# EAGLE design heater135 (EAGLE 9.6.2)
DATABASE: Z:\Eigene Dateien\Anwendungsdaten\Eagle\partdb\exp.txt
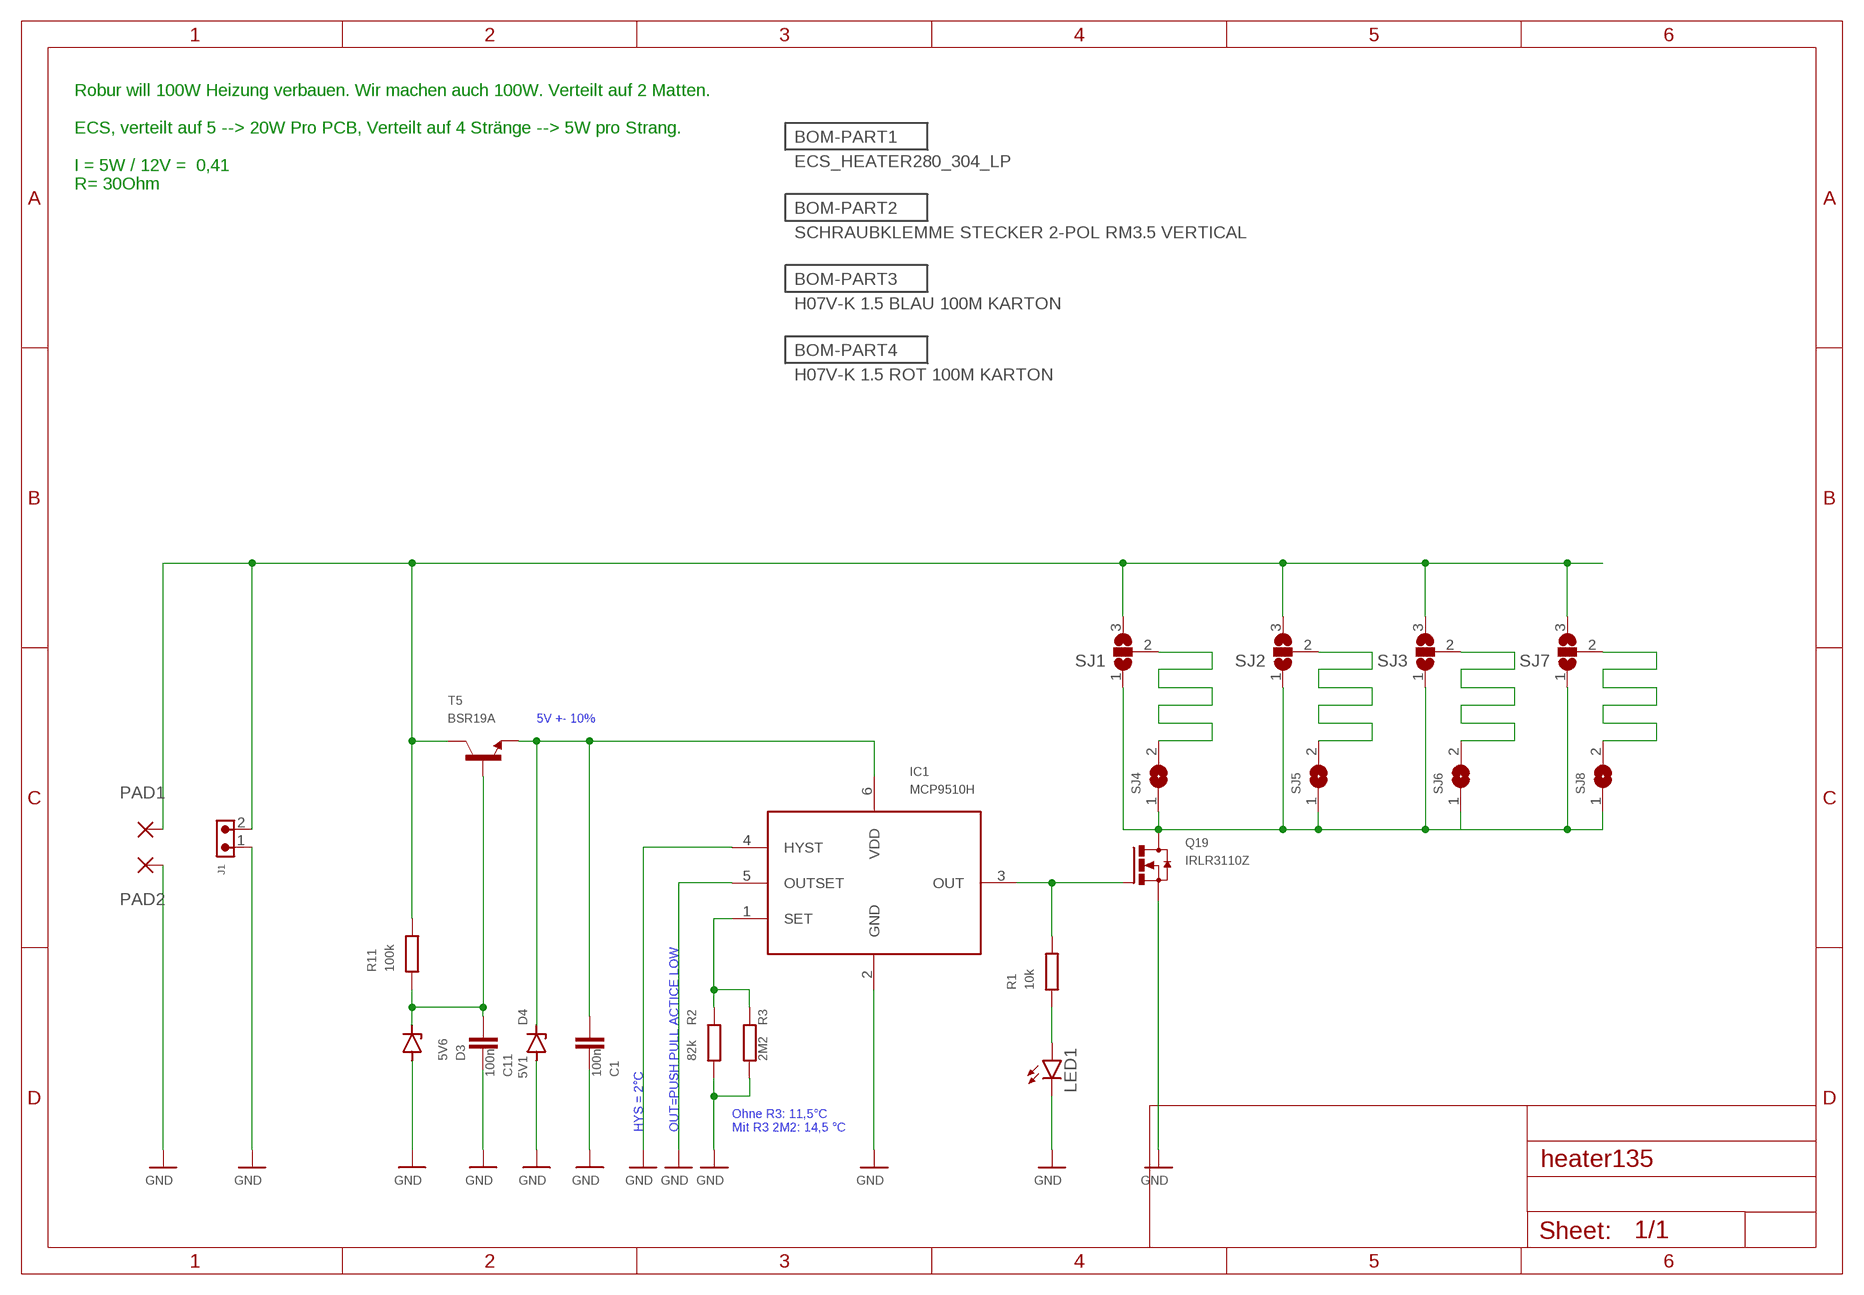
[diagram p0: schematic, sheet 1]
BOM-PART1 (BOM-PART): BOM: INCLUDE; PARTNO: PT055; QTY: 1
BOM-PART2 (BOM-PART): BOM: INCLUDE; PARTNO: CON181; QTY: 1
BOM-PART3 (BOM-PART): BOM: INCLUDE; QTY: 1
BOM-PART4 (BOM-PART): BOM: INCLUDE; QTY: 1

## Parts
C1  100n  C-EUC0603  [C0603]
C11  100n  C-EUC0603  [C0603]
D3  5V6  ZENER-DIODESOD80C  [SOD80C]
D4  5V1  ZENER-DIODESOD80C  [SOD80C]
IC1  MCP9510H  MCP9509  [SOT23-6]
J1  691322110002  [691322110002]
LED1  LEDSML0603  [SML0603]
PAD1  3,81/1,4  [3,81/1,4]
PAD2  3,81/1,4  [3,81/1,4]
Q19  IRLR3110Z  IRFR2607  [D-PACK]
R1  10k  R-EU_R0603  [R0603]
R2  82k  R-EU_R0603  [R0603]
R3  2M2  R-EU_R0603  [R0603]
R11  100k  R-EU_R0603  [R0603]
SJ1  SJ2W  [SJ_2]
SJ2  SJ2W  [SJ_2]
SJ3  SJ2W  [SJ_2]
SJ4  SJ  [SJ]
SJ5  SJ  [SJ]
SJ6  SJ  [SJ]
SJ7  SJ2W  [SJ_2]
SJ8  SJ  [SJ]
T5  BSR19A  MMBT2222ALT1-NPN-SOT23-BEC  [SOT23-BEC]

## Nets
+UB: J1.2 PAD1.1(P) R11.2 SJ1.3 SJ2.3 SJ3.3 SJ7.3 T5.C
GND: C1.2 C11.2 D3.A D4.A IC1.2(GND) IC1.4(HYST) IC1.5(OUTSET) J1.1 LED1.C PAD2.1(P) Q19.3(S) R2.1 R3.1
N$1: IC1.3(OUT) Q19.1(G) R1.2
N$2: SJ1.2 SJ4.2
N$3: C11.1 D3.C R11.1 T5.B
N$4: IC1.1(SET) R2.2 R3.2
N$5: C1.1 D4.C IC1.6(VDD) T5.E
N$6: LED1.A R1.1
N$7: SJ2.2 SJ5.2
N$8: SJ3.2 SJ6.2
N$9: SJ7.2 SJ8.2
N$11: Q19.4(D) SJ1.1 SJ2.1 SJ3.1 SJ4.1 SJ5.1 SJ6.1 SJ7.1 SJ8.1

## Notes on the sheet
- Robur will 100W Heizung verbauen. Wir machen auch 100W. Verteilt auf 2 Matten.
  
  ECS, verteilt auf 5 --> 20W Pro PCB, Verteilt auf 4 Stränge --> 5W pro Strang.
  
  I = 5W / 12V =  0,41
  R= 30Ohm
- 5V +- 10%
- HYS = 2°C | OUT=PUSH PULL ACTICE LOW
- Ohne R3: 11,5°C
  Mit R3 2M2: 14,5 °C

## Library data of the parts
C1 C11 = rcl:C-EU: CAPACITOR, European symbol; PARTNO: C067; SPICEPREFIX: C
D3 = diode:ZENER-DIODE: Z-Diode; PARTNO: D013
D4 = diode:ZENER-DIODE: Z-Diode; PARTNO: D012
IC1 = mcp9509:MCP9509; PARTNO: IC333
J1 = Wurth_Connectors_WR-TBL Pluggable Connector:691322110002: WR-TBL Serie 3221 - 3.50 mm Horizontal PCB Header; DATASHEET-URL: https://www.we-online.com/catalog/datasheet/691322110002.pdf; IR-UL: 10A; IR-VDE: 10.5A; MOUNT: THT; PART-NUMBER: 691322110002; PARTNO: CON212; PINS: 2; PITCH: 3.5mm; TYPE: Horizontal; WORKING-VOLTAGE-UL: 300V (AC); WORKING-VOLTAGE-VDE: 300V (AC)
LED1 = led:LED: LED; PARTNO: D078
PAD1 PAD2 = wirepad:3,81/1,4: THROUGH-HOLE PAD
Q19 = IRFR2607:IRFR2607; PARTNO: T086
R1 = rcl:R-EU_: RESISTOR, European symbol; PARTNO: R221; SPICEPREFIX: R
R2 = rcl:R-EU_: RESISTOR, European symbol; PARTNO: R243; SPICEPREFIX: R
R3 = rcl:R-EU_: RESISTOR, European symbol; PARTNO: R277; SPICEPREFIX: R
R11 = rcl:R-EU_: RESISTOR, European symbol; PARTNO: R245; SPICEPREFIX: R
SJ1-SJ3 SJ7 = jumper:SJ2W: SMD solder JUMPER
SJ4-SJ6 SJ8 = jumper:SJ: SMD solder JUMPER
T5 = transistor-neu-to92:*-NPN-: NPN Transistror; PARTNO: T056

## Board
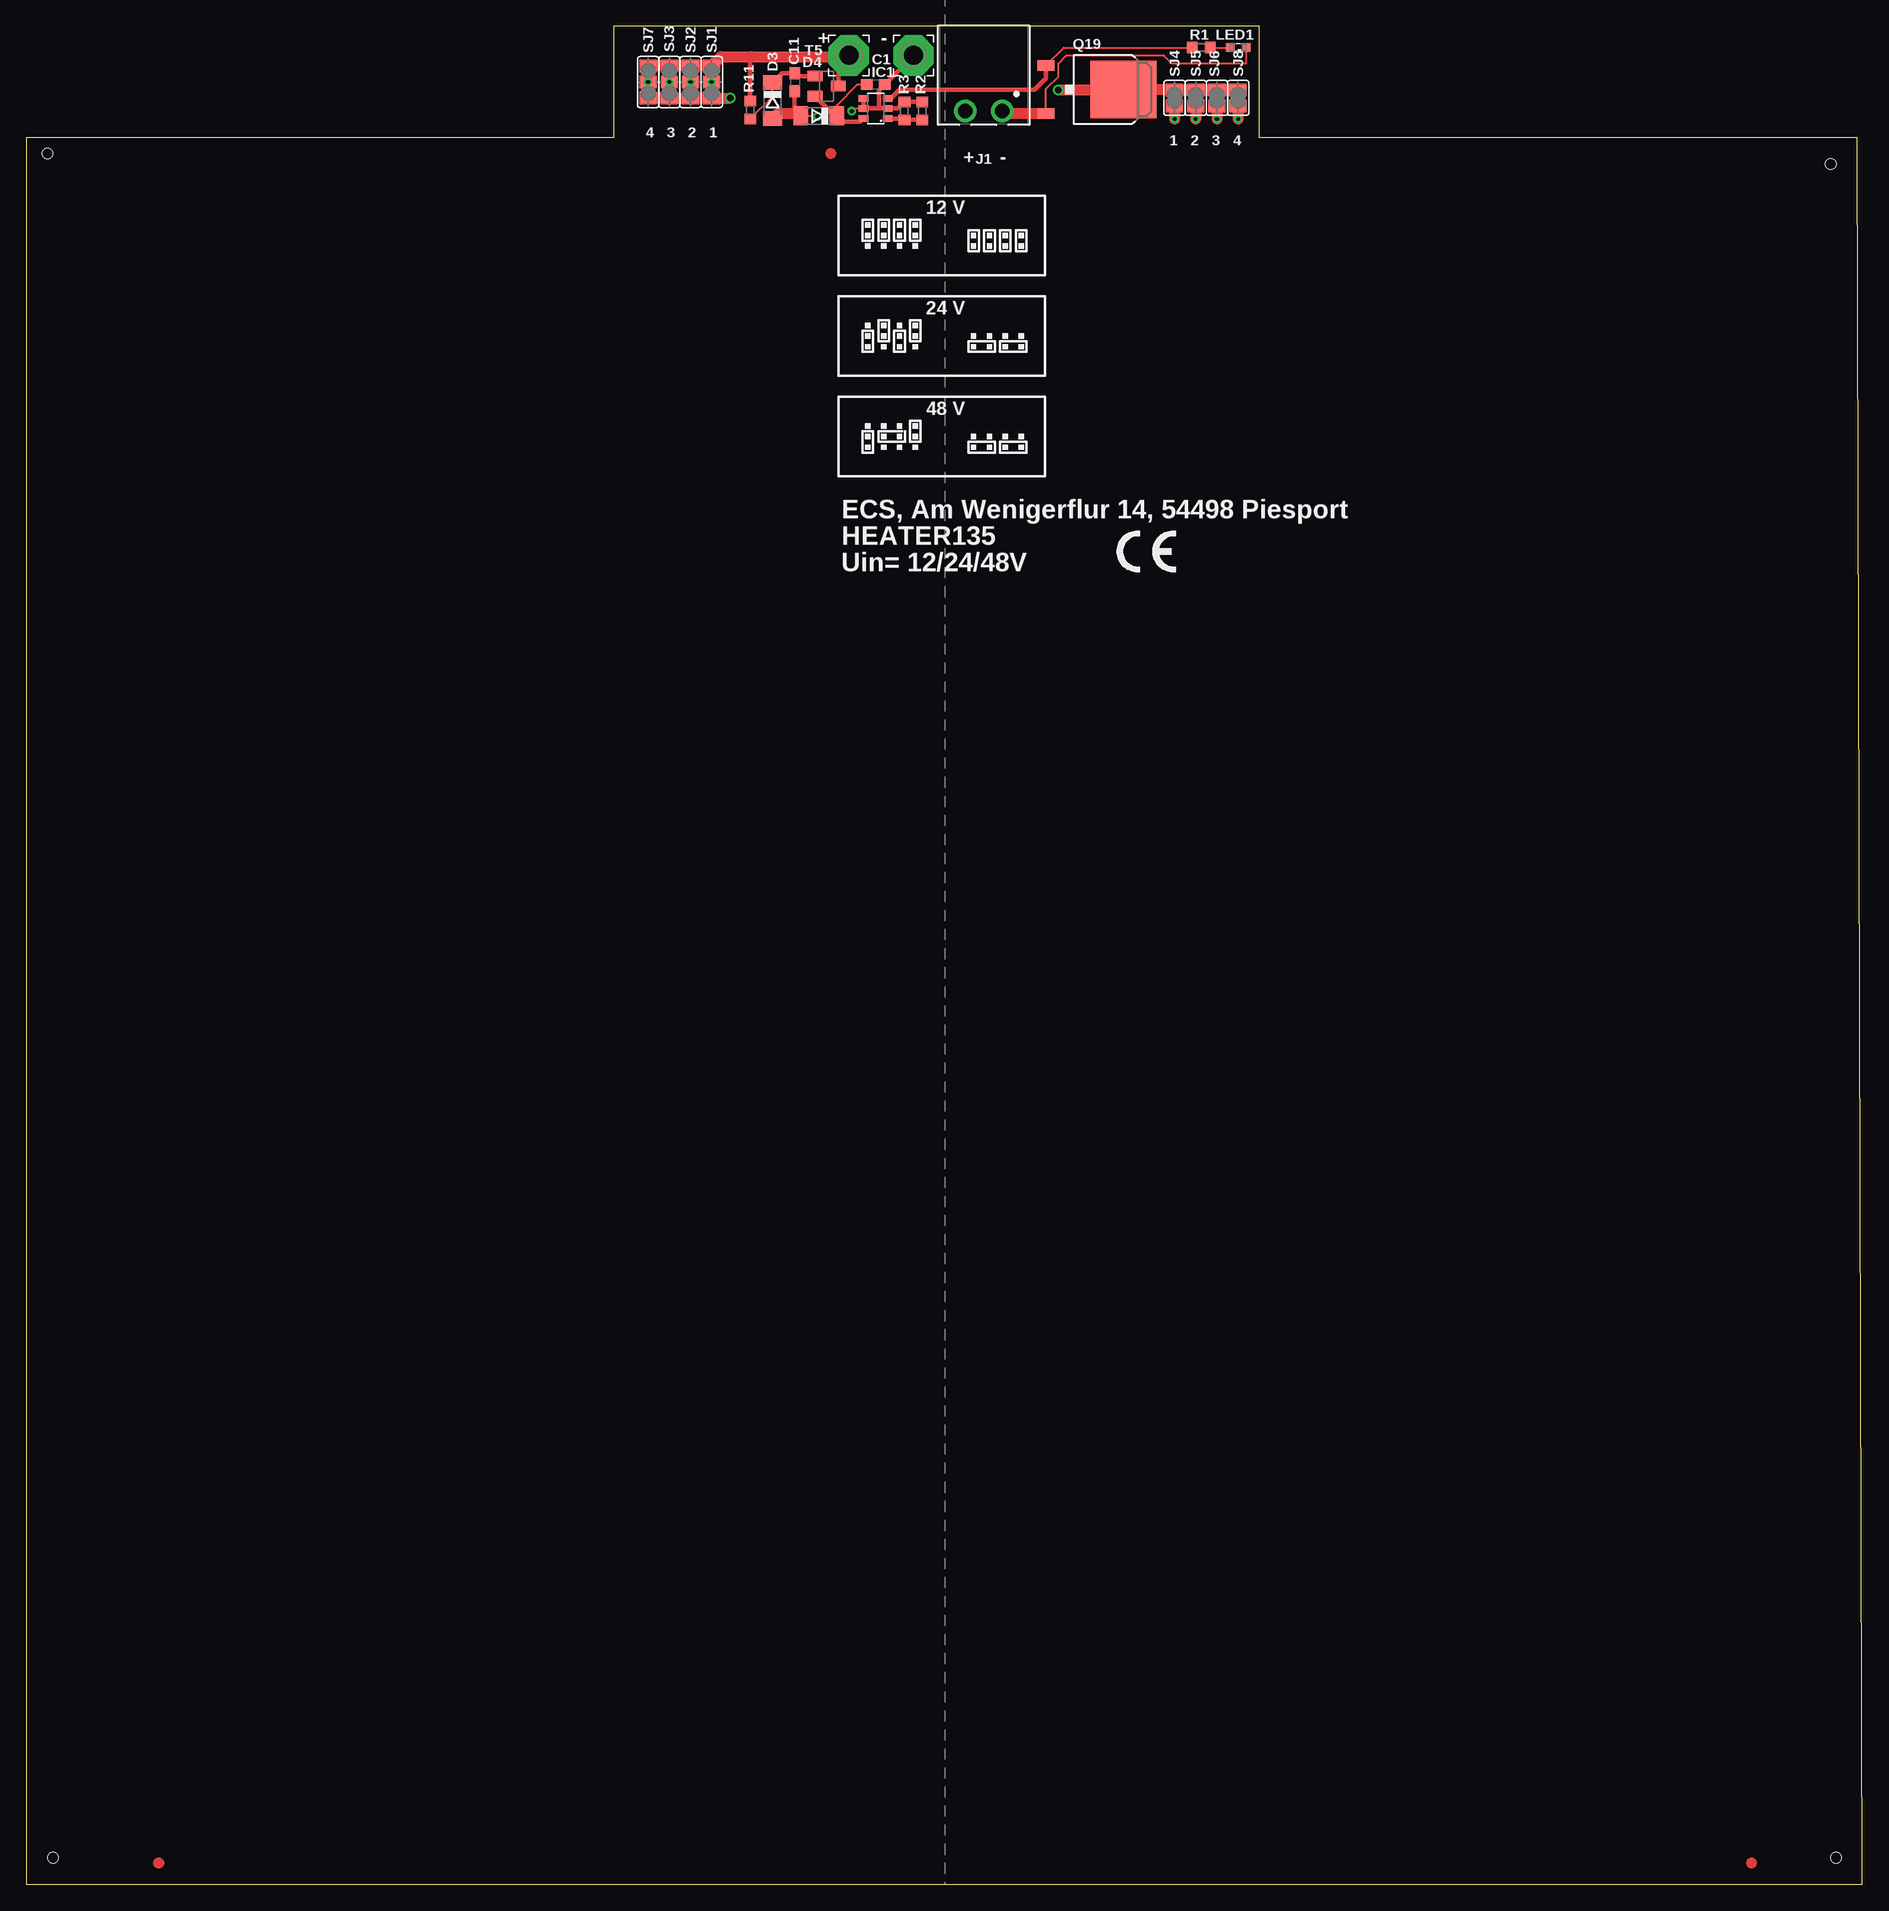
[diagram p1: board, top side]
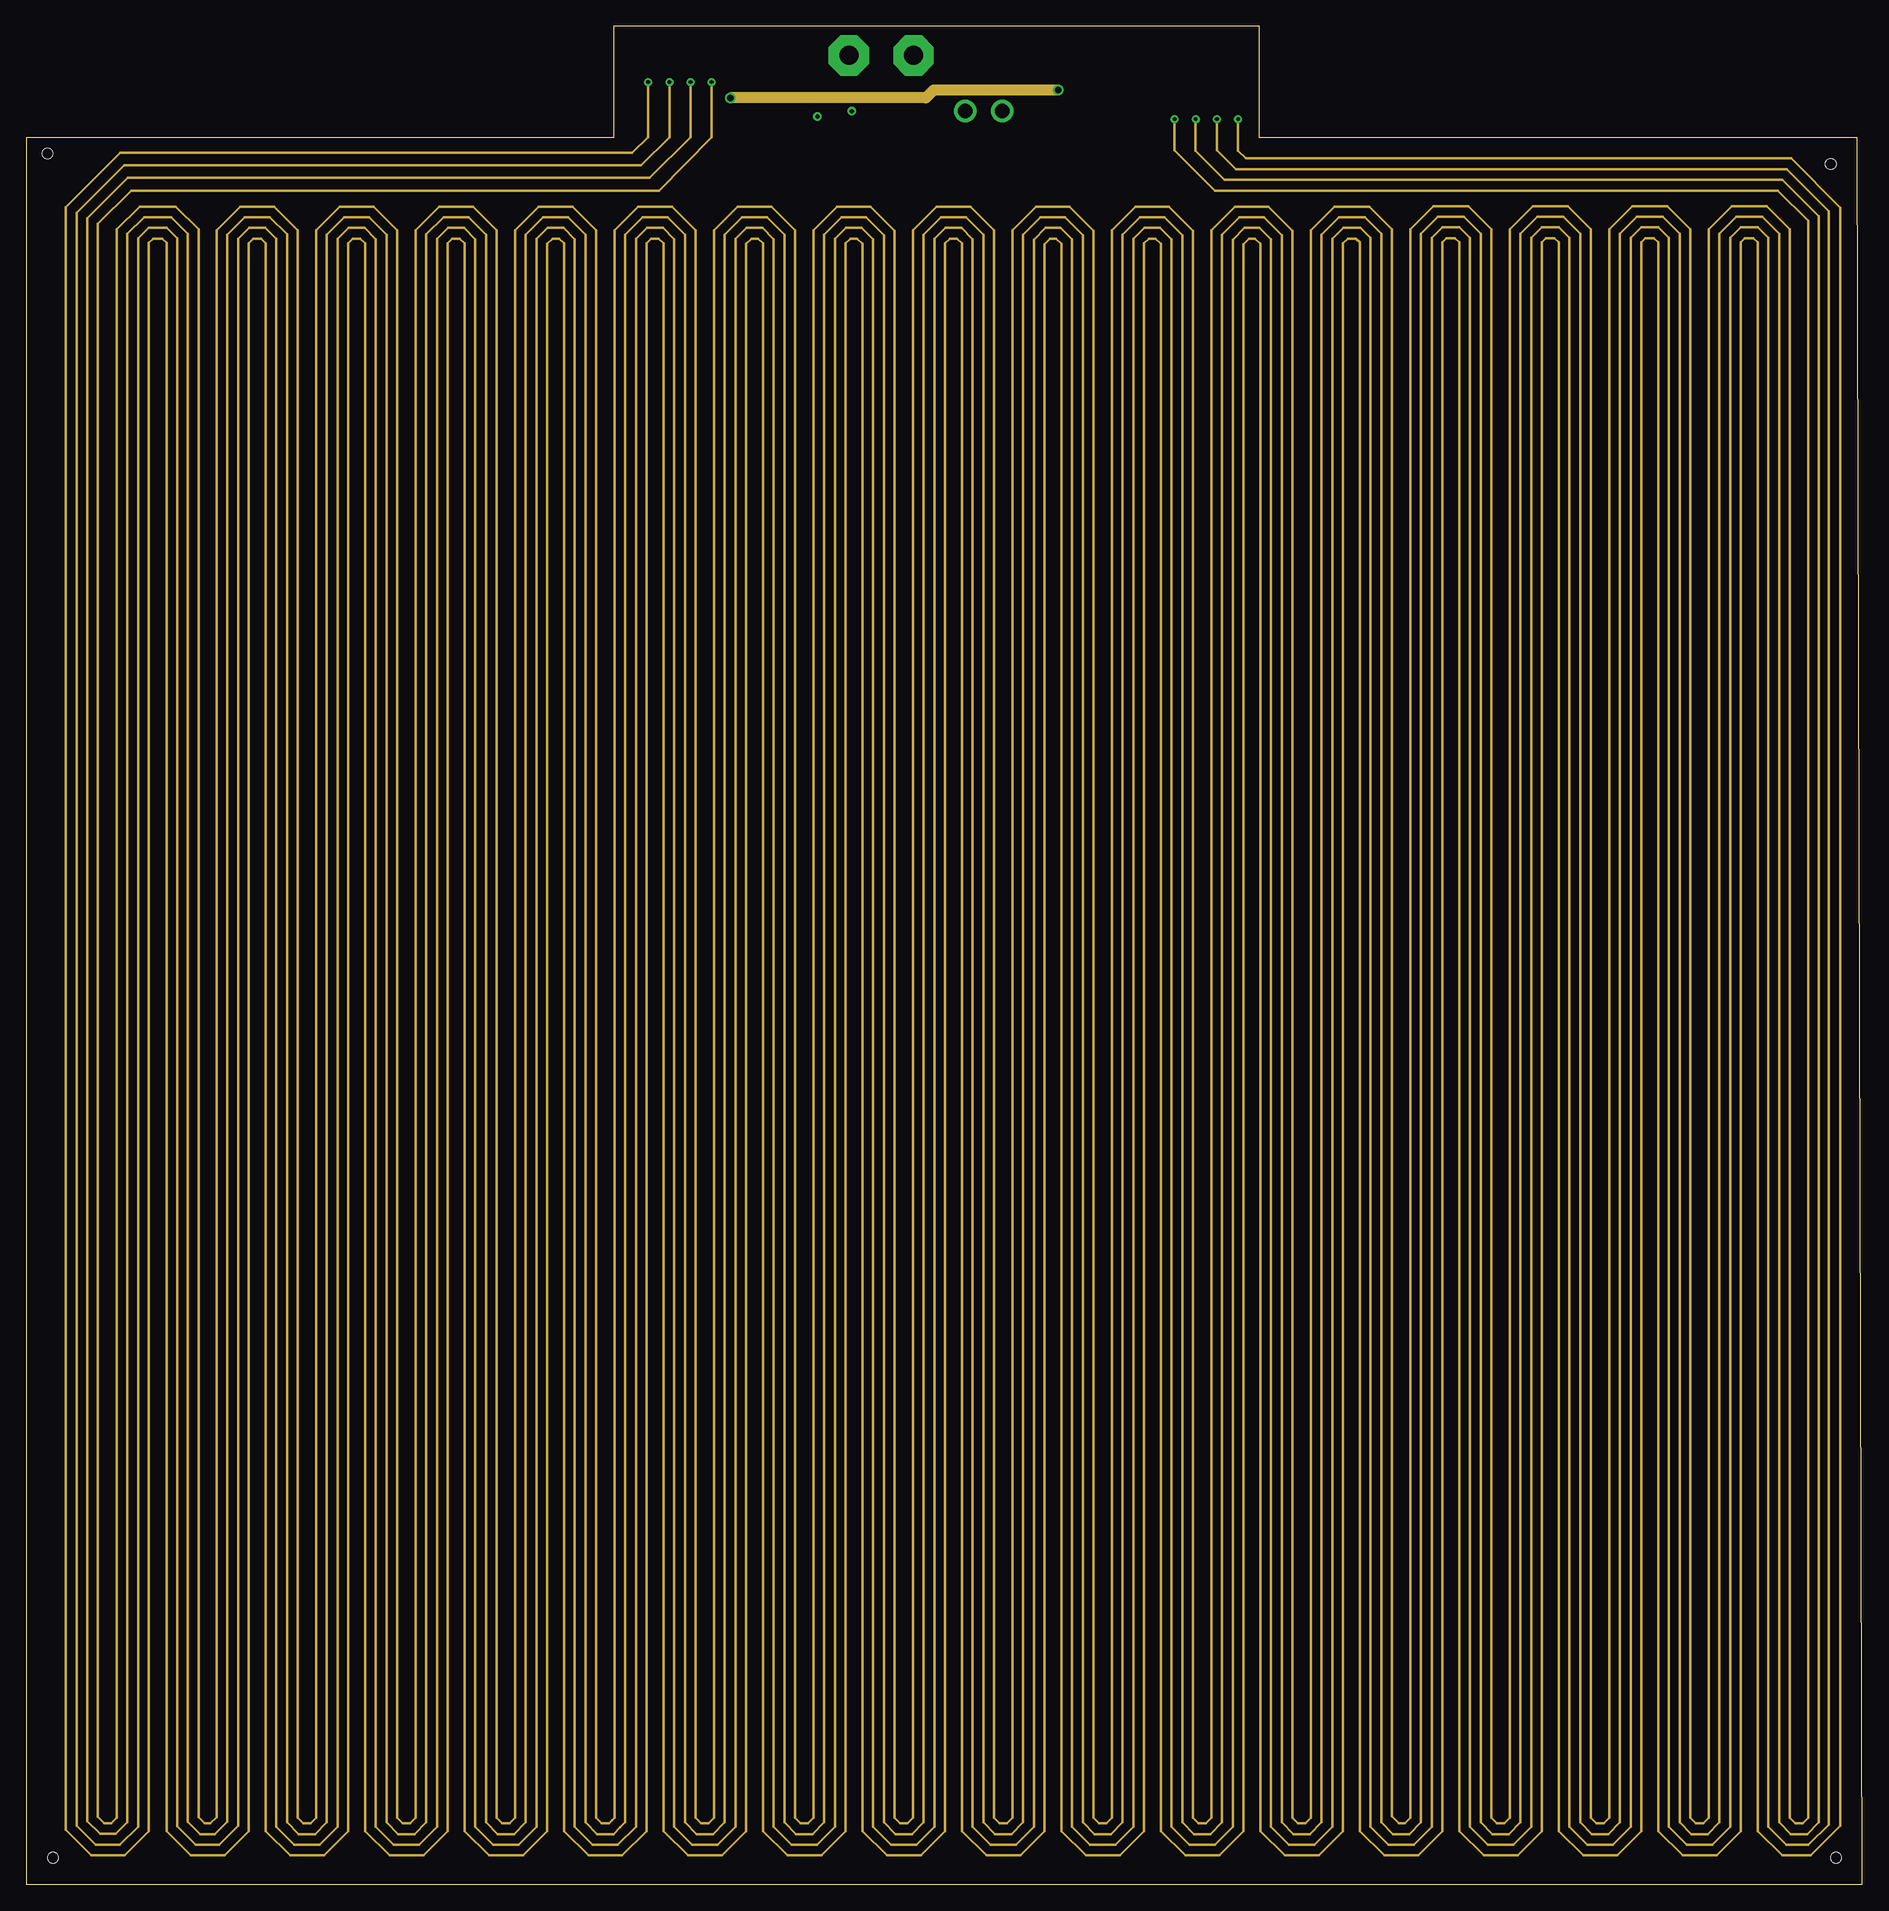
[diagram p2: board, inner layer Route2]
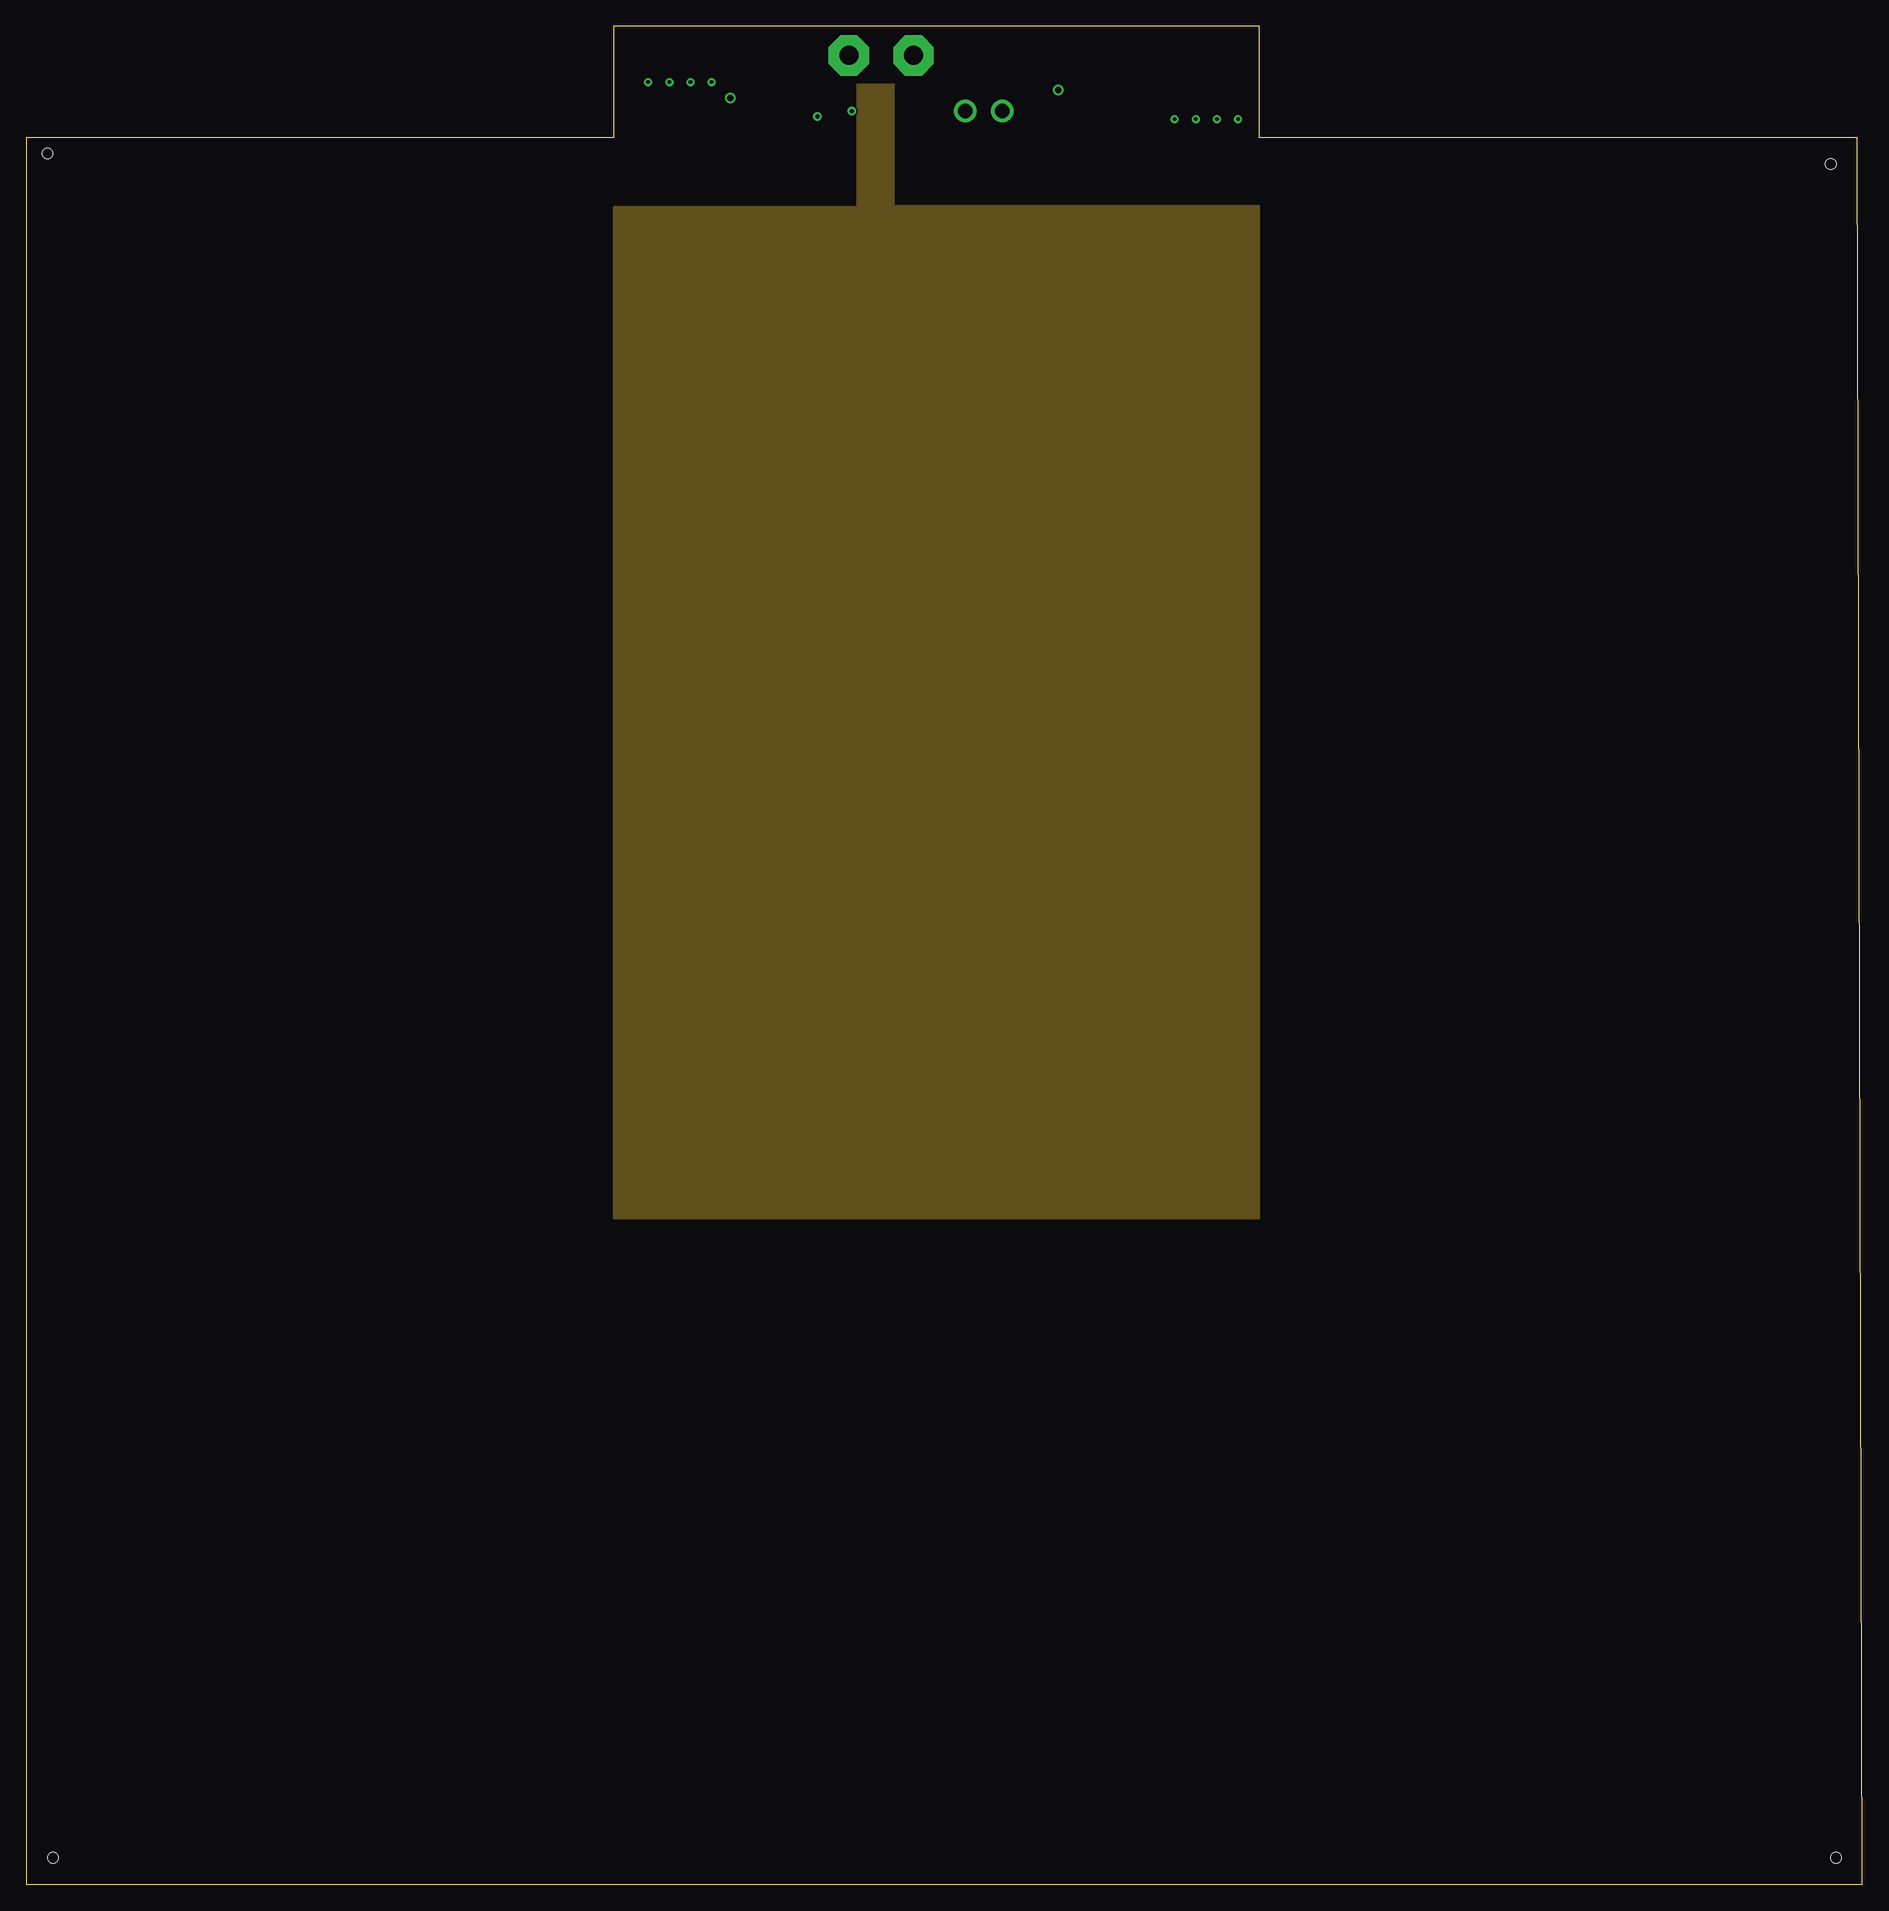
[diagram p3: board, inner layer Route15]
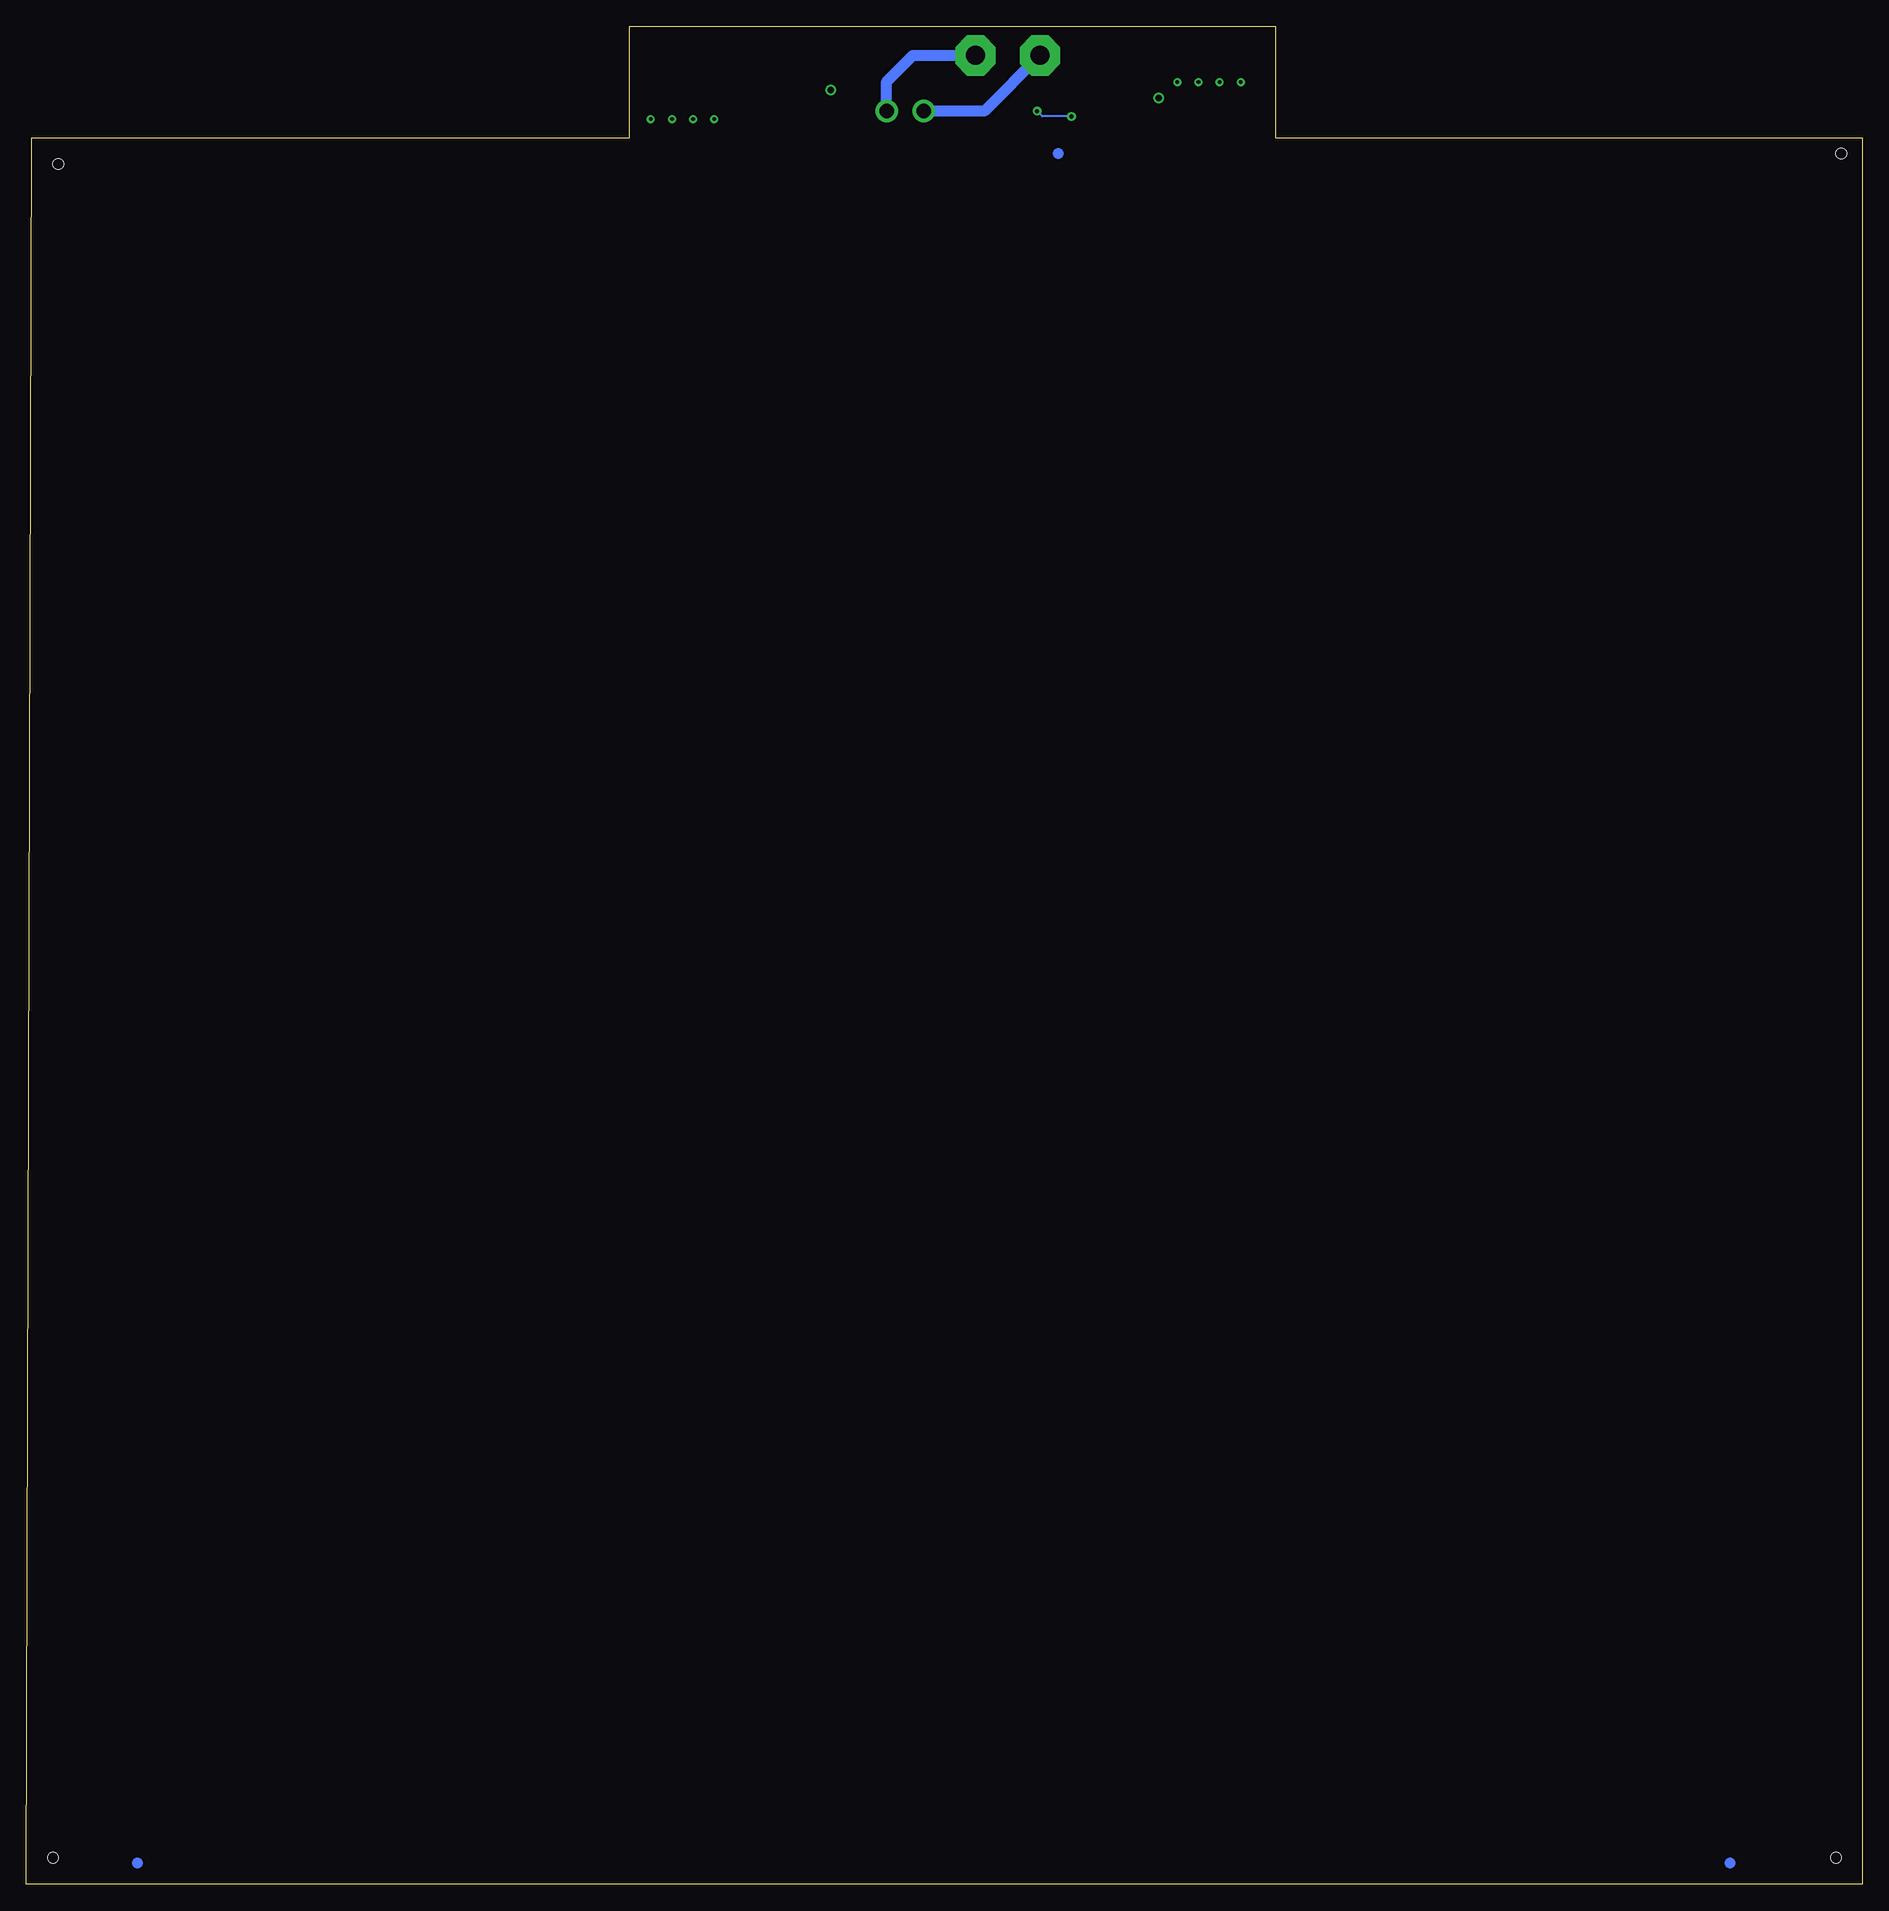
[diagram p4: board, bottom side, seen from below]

Size 173.5 x 175.5 mm. Coordinates in mm from the lower left corner, seen from the top.
Outline: 0,0 173.5,0 173,165 116.5,165 116.5,175.5 55.5,175.5 55.5,165 0,165 0,0
Copper layers (1+2*15+16): Top 0.035mm / dielectric 1.5mm / Route2 0.0175mm / dielectric 0.15mm / Route15 0.0175mm / dielectric 0.2mm / Bottom 0.035mm
Design rules "default *": minimum track width 6mil, minimum drill 0.35mm, track to track 6mil, track to pad 6mil, pad to pad 6mil, via to via 6mil, smd to smd 6mil, copper to edge 40mil, drill to drill 6mil, minimum pad ring 10mil, minimum via ring 8mil, stop-mask expansion 4mil, vias tented up to drill 0mil, thermal gap 10mil
Holes 1 mm at 2,163.5 170.5,162.5 171,2.5 2.5,2.5

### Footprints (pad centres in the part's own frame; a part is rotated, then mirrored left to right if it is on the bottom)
C0603 = smd 1.1 x 1: 1 -0.85,0; 2 0.85,0
SOD80C = smd 1.4 x 1.8: A 1.7,0; C -1.7,0
SOT23-6 = smd 0.6 x 0.9: 1 -0.95,-1.15; 2 0,-1.15; 3 0.95,-1.15; 4 0.95,1.15; 5 0,1.15; 6 -0.95,1.15
691322110002 = drill 1.4: 1 -1.75,0; 2 1.75,0
SML0603 = smd 0.8 x 0.8: A 0.75,0; C -0.75,0
3,81/1,4 = drill 1.8 pad 3.81 octagon: 1 0,0
D-PACK = smd 1 x 1.6: 1 -2.28,-4.8; 3 2.28,-4.8 | smd 5.4 x 6.2: 4 0,2.5
R0603 = smd 1 x 1.1: 1 -0.85,0; 2 0.85,0
SJ_2 = smd 1.168 x 1.6: 1 -1.524,0; 2 0,0; 3 1.524,0
SJ = smd 1.168 x 1.6: 1 -0.762,0; 2 0.762,0
SOT23-BEC = smd 1 x 1.4: B -0.95,-1.1; C 0,1.1; E 0.95,-1.1

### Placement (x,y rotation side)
C1  80.27,170.02 0 top
C11  72.6,170.23 270 top
D3  70.5,168.5 270 top
D4  74.88,167.05 180 top
IC1  80.25,167.75 90 top
J1  90.46,167.51 180 top
LED1  114.5,173.5 180 top
PAD1  77.72,172.76 0 top
PAD2  83.82,172.76 0 top
Q19  101.16,169.55 270 top
R1  111,173.5 180 top
R2  84.64,167.52 270 top
R3  82.97,167.52 270 top
R11  68.4,167.62 90 top
SJ1  64.75,170.25 90 top
SJ2  62.75,170.25 90 top
SJ3  60.75,170.25 90 top
SJ4  108.5,168.75 270 top
SJ5  110.5,168.75 270 top
SJ6  112.5,168.75 270 top
SJ7  58.75,170.25 90 top
SJ8  114.5,168.75 270 top
T5  75.61,169.86 270 top
U$1  [CE-4MM]  103,123.88 0 top
U$2  [CIRCLE-1MM-3R]  12.5,2 0 top
U$3  [CIRCLE-1MM-3R]  163,2 0 top
U$4  [CIRCLE-1MM-3R]  76,163.5 0 top

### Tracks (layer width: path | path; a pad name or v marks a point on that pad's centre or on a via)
+UB
  Top 0.406: T5.C 76.75,169.9 76.75,171.79 77.61,172.65 PAD1.1 | R11.2 68.4,172.54 68.5,172.65
  Top 1.016: SJ7.3 SJ3.3 SJ2.3 SJ1.3 65.62,172.65 68.5,172.65 77.61,172.65
  Bottom 1.016: PAD1.1 82.97,167.51 J1.2
GND  (via drill 0.4)
  Top 0.2: LED1.C 115.25,172 108.25,172 107.5,172.75 98.25,172.75 97.5,172 97.5,170.75 96.36,169.61 Q19.3 | D4.A 74.7,167.05 v74.75,167 | v78,167.5 78.25,167.75 IC1.5
  Top 0.406: D4.A 72.6,167.63 C11.2 | 80.56,167.75 IC1.2 82.35,167.75 R3.1 R2.1 | 80.56,167.75 80.56,169.46 C1.2 81.12,170.06 PAD2.1 | IC1.4 IC1.5 80.56,167.75
  Top 1.016: D3.A 70.95,167.25 72.98,167.25 D4.A | Q19.3 92.45,167.27 J1.1
  Bottom 0.2: v74.75,167 77.5,167 v78,167.5
  Bottom 1.016: J1.1 92.21,170.29 89.74,172.76 PAD2.1
N$1
  Top 0.2: Q19.1 98.03,173.5 R1.2
  Top 0.406: IC1.3 81.7,168.7 82.5,169.5 95.25,169.5 96.36,170.61 Q19.1
N$2  (via drill 0.35, 0.35 pad 0.21)
  Top 1.016: SJ4.2 v108.5,166.75
  Route2 0.254: SJ1.2 64.75,165.02 59.79,160 9.9,160 6.75,156.85 6.75,6.37 7.37,5.76 8.01,5.76 8.54,6.28 8.54,156.32 10.71,158.49 14.09,158.49 16.26,156.32 16.26,6.32 16.84,5.75 17.38,5.75 17.97,6.34 17.97,156.26 20.2,158.49 23.41,158.49 25.63,156.27 25.63,6.27 26.16,5.75 26.86,5.75 27.37,6.25 27.37,156.26 29.6,158.49 32.79,158.49 35.03,156.25 35.03,6.27 35.55,5.75 36.26,5.75 36.77,6.25 36.77,156.27 38.99,158.49 42.19,158.49 44.43,156.25 44.43,6.27 44.95,5.75 45.66,5.75 46.17,6.25 46.17,156.26 48.4,158.49 51.59,158.49 53.83,156.25 53.83,6.27 54.35,5.75 55.05,5.75 55.35,6.05 55.57,6.27 55.57,156.26 57.8,158.49 60.99,158.49 63.23,156.25 63.23,6.27 63.75,5.75 64.47,5.75 64.97,6.25 64.97,156.26 67.2,158.49 70.39,158.49 72.63,156.25 72.63,6.27 73.16,5.75 73.86,5.75 74.37,6.25 74.37,156.26 76.6,158.49 79.75,158.49 82.03,156.22 82.03,6.27 82.56,5.75 83.26,5.75 83.77,6.25 83.77,156.26 86,158.49 89.19,158.49 91.43,156.25 91.43,6.27 91.95,5.75 92.66,5.75 93.17,6.25 93.17,156.26 95.4,158.49 98.56,158.49 100.83,156.22 100.83,6.27 101.35,5.75 102.07,5.75 102.57,6.25 102.57,156.26 104.8,158.49 107.95,158.49 110.23,156.22 110.23,6.27 110.75,5.75 111.46,5.75 111.97,6.25 111.97,156.26 114.2,158.49 117.36,158.49 119.63,156.22 119.63,6.27 120.16,5.75 120.86,5.75 121.37,6.25 121.37,156.26 123.6,158.49 126.89,158.49 129.03,156.35 129.03,6.42 129.7,5.75 130.26,5.75 130.77,6.25 130.77,156.35 132.94,158.53 136.25,158.53 138.43,156.35 138.43,6.27 138.96,5.75 139.66,5.75 140.17,6.25 140.17,156.35 142.34,158.53 145.66,158.53 147.83,156.35 147.83,6.27 148.35,5.75 149.06,5.75 149.57,6.25 149.57,156.35 151.75,158.53 155.06,158.53 157.23,156.35 157.23,6.27 157.75,5.75 158.46,5.75 158.97,6.25 158.97,156.35 161.15,158.53 164.46,158.53 166.63,156.35 166.63,6.27 167.16,5.75 167.86,5.75 168.37,6.25 168.37,157.13 165.5,160 112.3,160 108.5,163.8 v108.5,166.75
  other vias: 64.75,170.25
N$3
  Top 0.2: R11.1 70.5,168.87 D3.C
  Top 0.406: D3.C 71.38,171.08 C11.1 72.87,170.81 T5.B
N$4
  Top 0.406: IC1.1 82.97,166.8 R3.2 R2.2
N$5
  Top 0.2: C1.1 79.4,170 78.5,170 76.58,168.08 D4.C
  Top 0.406: T5.E 76.37,167.05 D4.C 76.83,166.8 76.95,166.8 77.25,166.5 78.77,166.5 IC1.6
N$6
  Top 0.2: R1.1 LED1.A
N$7  (via drill 0.35, 0.35 pad 0.21)
  Top 1.016: SJ5.2 v110.5,166.75
  Route2 0.254: SJ2.2 62.75,165.05 58.9,161.2 9.56,161.2 5.74,157.39 5.74,5.95 6.95,4.75 8.43,4.75 9.54,5.86 9.54,155.9 11.13,157.48 13.67,157.48 15.26,155.9 15.26,5.9 16.42,4.74 17.8,4.74 18.98,5.92 18.98,155.84 20.62,157.48 22.99,157.48 24.62,155.85 24.62,5.85 25.74,4.74 27.28,4.74 28.38,5.84 28.38,155.84 30.02,157.48 32.38,157.48 34.02,155.84 34.02,5.85 35.14,4.74 36.68,4.74 37.78,5.84 37.78,155.85 39.41,157.48 41.77,157.48 43.42,155.84 43.42,5.85 44.54,4.74 46.08,4.74 47.18,5.84 47.18,155.84 48.82,157.48 51.17,157.48 52.82,155.84 52.82,5.85 53.93,4.74 55.47,4.74 56.12,5.38 56.58,5.85 56.58,155.84 58.22,157.48 60.57,157.48 62.22,155.84 62.22,5.85 63.34,4.74 64.88,4.74 65.98,5.84 65.98,155.84 67.62,157.48 69.97,157.48 71.62,155.84 71.62,5.85 72.74,4.74 74.28,4.74 75.38,5.84 75.38,155.84 77.02,157.48 79.34,157.48 81.02,155.8 81.02,5.85 82.14,4.74 83.68,4.74 84.78,5.84 84.78,155.84 86.42,157.48 88.77,157.48 90.42,155.84 90.42,5.85 91.54,4.74 93.08,4.74 94.18,5.84 94.18,155.84 95.82,157.48 98.14,157.48 99.82,155.8 99.82,5.85 100.94,4.74 102.48,4.74 103.58,5.84 103.58,155.84 105.22,157.48 107.54,157.48 109.22,155.8 109.22,5.85 110.34,4.74 111.88,4.74 112.98,5.84 112.98,155.84 114.62,157.48 116.94,157.48 118.62,155.8 118.62,5.85 119.74,4.74 121.28,4.74 122.38,5.84 122.38,155.84 124.02,157.48 126.47,157.48 128.02,155.94 128.02,5.85 129.14,4.74 130.68,4.74 131.78,5.84 131.78,155.94 133.36,157.52 135.84,157.52 137.42,155.94 137.42,5.85 138.54,4.74 140.08,4.74 141.18,5.84 141.18,155.94 142.76,157.52 145.24,157.52 146.82,155.94 146.82,5.85 147.94,4.74 149.48,4.74 150.58,5.84 150.58,155.94 152.16,157.52 154.64,157.52 156.22,155.94 156.22,5.85 157.34,4.74 158.88,4.74 159.98,5.84 159.98,155.94 161.56,157.52 164.04,157.52 165.62,155.94 165.62,5.85 166.74,4.74 168.28,4.74 169.38,5.84 169.38,157.55 165.92,161.01 113.22,161.01 110.46,163.76 110.46,166.71
  Route2 0.4: 110.46,166.71 v110.5,166.75
  other vias: 62.75,170.25
N$8  (via drill 0.35, 0.35 pad 0.21)
  Top 1.016: SJ6.2 v112.5,166.75
  Route2 0.254: SJ3.2 60.75,165.05 58.1,162.4 9.23,162.4 4.74,157.91 4.74,5.53 6.54,3.73 8.84,3.73 10.55,5.45 10.55,155.48 11.54,156.47 13.26,156.47 14.24,155.48 14.24,5.48 16,3.73 18.22,3.73 19.99,5.5 19.99,155.43 21.04,156.47 22.57,156.47 23.61,155.44 23.61,5.43 25.32,3.73 27.7,3.73 29.39,5.42 29.39,155.43 30.43,156.47 31.96,156.47 33.01,155.42 33.01,5.43 34.72,3.73 37.1,3.73 38.79,5.42 38.79,155.44 39.83,156.47 41.36,156.47 42.41,155.42 42.41,5.43 44.12,3.73 46.5,3.73 48.19,5.42 48.19,155.43 49.24,156.47 50.76,156.47 51.81,155.42 51.81,5.43 53.52,3.73 55.88,3.73 57.59,5.43 57.59,155.43 58.64,156.47 60.16,156.47 61.21,155.42 61.21,5.43 62.92,3.73 65.3,3.73 66.99,5.42 66.99,155.43 68.04,156.47 69.56,156.47 70.61,155.42 70.61,5.43 72.32,3.73 74.7,3.73 76.39,5.42 76.39,155.43 77.44,156.47 78.92,156.47 80.01,155.38 80.01,5.43 81.72,3.73 84.1,3.73 85.79,5.42 85.79,155.43 86.84,156.47 88.36,156.47 89.41,155.42 89.41,5.43 91.12,3.73 93.5,3.73 95.19,5.42 95.19,155.36 96.3,156.47 97.72,156.47 98.81,155.38 98.81,5.43 100.52,3.73 102.9,3.73 104.59,5.42 104.59,155.43 105.64,156.47 107.12,156.47 108.21,155.38 108.21,5.43 109.92,3.73 112.3,3.73 113.99,5.42 113.99,155.36 115.1,156.47 116.52,156.47 117.61,155.38 117.61,5.43 119.32,3.73 121.7,3.73 123.39,5.42 123.39,155.43 124.44,156.47 126.06,156.47 127.01,155.52 127.01,5.43 128.72,3.73 131.1,3.73 132.79,5.42 132.79,155.52 133.78,156.51 135.42,156.51 136.41,155.52 136.41,5.43 138.12,3.73 140.5,3.73 142.19,5.42 142.19,155.52 143.18,156.51 144.82,156.51 145.81,155.52 145.81,5.43 147.52,3.73 149.9,3.73 151.59,5.42 151.59,155.52 152.58,156.51 154.22,156.51 155.21,155.52 155.21,5.43 156.92,3.73 159.3,3.73 160.99,5.42 160.99,155.52 161.98,156.51 163.62,156.51 164.61,155.52 164.61,5.43 166.32,3.73 168.4,3.73 170.29,5.62 170.29,158.06 166.34,162.02 114.28,162.02 112.5,163.8 v112.5,166.75
  other vias: 60.75,170.25
N$9  (via drill 0.35, 0.35 pad 0.21)
  Top 1.016: SJ8.2 v114.5,166.75
  Route2 0.254: SJ7.2 58.75,165.05 57.25,163.55 8.85,163.55 3.73,158.43 3.73,5.12 6.12,2.72 9.29,2.72 11.56,4.99 11.56,155.06 11.96,155.46 12.84,155.46 13.24,155.06 13.24,4.98 15.5,2.72 18.72,2.72 21,5 21,155.01 21.45,155.45 22.16,155.45 22.6,155.02 22.6,5.02 24.9,2.72 28.12,2.72 30.4,5 30.4,155.01 30.85,155.45 31.55,155.45 32,155 32,5.02 34.3,2.72 37.52,2.72 39.8,5 39.8,155.02 40.24,155.46 40.94,155.46 41.4,155 41.4,5.02 43.7,2.72 46.92,2.72 49.2,5 49.2,154.96 49.7,155.46 50.34,155.46 50.8,155 50.8,5 53.1,2.72 56.3,2.72 58.6,5 58.6,155.01 59.05,155.45 59.75,155.45 60.2,155 60.2,5.02 62.5,2.72 65.72,2.72 68,5 68,154.96 68.5,155.46 69.14,155.46 69.6,155 69.6,5.02 71.9,2.72 75.12,2.72 77.4,5 77.4,155.01 77.86,155.46 78.5,155.46 79,154.96 79,5.02 81.3,2.72 84.52,2.72 86.8,5 86.8,155.01 87.25,155.46 87.94,155.46 88.4,155 88.4,5.02 90.7,2.72 93.92,2.72 96.2,5 96.2,154.94 96.72,155.46 97.3,155.46 97.8,154.96 97.8,5.02 100.1,2.72 103.32,2.72 105.6,5 105.6,155.01 106.06,155.46 106.7,155.46 107.2,154.96 107.2,5.02 109.5,2.72 112.72,2.72 115,5 115,154.94 115.52,155.46 116.1,155.46 116.6,154.96 116.6,5.02 118.9,2.72 122.12,2.72 124.4,5 124.4,155.01 124.86,155.46 125.64,155.46 126,155.1 126,5.02 128.3,2.72 131.52,2.72 133.8,5 133.8,155.1 134.2,155.5 135,155.5 135.4,155.1 135.4,5.02 137.7,2.72 140.92,2.72 143.2,5 143.2,155.1 143.6,155.5 144.4,155.5 144.8,155.1 144.8,5.02 147.1,2.72 150.32,2.72 152.6,5 152.6,155.1 153,155.5 153.8,155.5 154.2,155.1 154.2,5.02 156.5,2.72 159.72,2.72 162,5 162,155.1 162.4,155.5 163.2,155.5 163.6,155.1 163.6,5.02 165.9,2.72 168.62,2.72 171.4,5.5 171.4,158.38 166.75,163.03 115.22,163.03 114.5,163.75 v114.5,166.75
  other vias: 58.75,170.25
N$10
  pour Route15: 78.5,170 78.5,158.4 55.5,158.4 55.5,62.9 116.5,62.9 116.5,158.5 82,158.5 82,170
N$11  (via drill 0.6)
  Top 1.016: SJ7.1 SJ3.1 SJ2.1 SJ1.1 66.48,168.73 v66.5,168.75 | SJ8.1 SJ6.1 SJ5.1 SJ4.1 104.65,169.51 103.66,170.5 Q19.4 103.61,169.5 v97.5,169.5
  Route2 1.016: v66.5,168.75 85,168.75 85.75,169.5 v97.5,169.5

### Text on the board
tPlace: + | - | 4 | 3 | 2 | 1 | 1 | 2 | 3 | 4 | + | - | 12 V | 24 V | 48 V | ECS, Am Wenigerflur 14, 54498 Piesport | HEATER135 | Uin= 12/24/48V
